PROGRAM MAIN
VAR
	Mode: INT := 1;
	bConnect: BOOL;
END_VAR

stComSerialCfg.Baudrate := 19200;
stComSerialCfg.ComPort 	:= 1;
stComSerialCfg.DataBits := 8;
stComSerialCfg.StopBits := Tc2_SerialCom.STOPBITS_ONE;
stComSerialCfg.Parity 	:= Tc2_SerialCom.PARITY_NONE;
fbUSBSerial(
	Connect:= bConnect, 
	SerialCfg:= stComSerialCfg, 
	NetId:= '', 
	Timeout:= T#1S, 
	TxBuffer:= TxBuffer, 
	RxBuffer:= RxBuffer, 
	PortOpened=> , 
	Error=> , 
	ErrorID=> , 
	Busy=> , 
	TxBufCount=> , 
	RxBufCount=> );
IF fbUSBSerial.PortOpened THEN
	CASE Mode OF
		1:ModbusRTU_Master();	// Test with Modsim
		2:ModbusRTU_Slave();	// Test with Modscan
		3:SerialCom();			// Test with JCom
	END_CASE
END_IF

END_PROGRAM
